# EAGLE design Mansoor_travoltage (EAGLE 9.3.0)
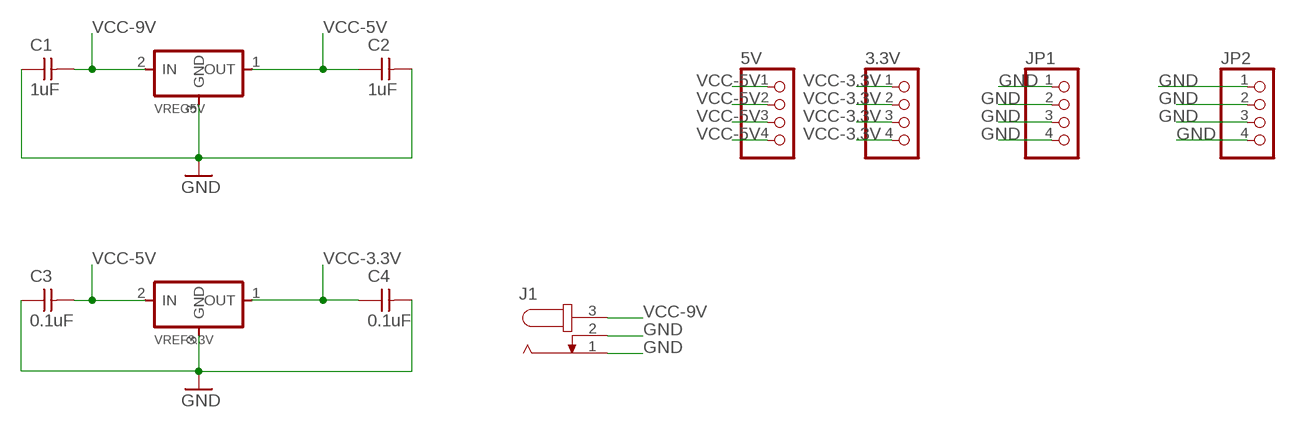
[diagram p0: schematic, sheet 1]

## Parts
3.3V  PINHD-1X4/LONG  [1X04]
5V  PINHD-1X4/LONG  [1X04]
C1  1uF  CAP-UNPOLARIZEDFAB  [C1206FAB]
C2  1uF  CAP-UNPOLARIZEDFAB  [C1206FAB]
C3  0.1uF  CAP-UNPOLARIZEDFAB  [C1206FAB]
C4  0.1uF  CAP-UNPOLARIZEDFAB  [C1206FAB]
J1  JACK-PLUG1  [SPC4078]
JP1  PINHD-1X4/LONG  [1X04]
JP2  PINHD-1X4/LONG  [1X04]
VREF3.3V  REGULATORSOT23  [SOT23]
VREG5V  REGULATORSOT23  [SOT23]

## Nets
GND: C1.1 C2.2 C3.1 C4.2 J1.1 J1.2 JP1.1 JP1.2 JP1.3 JP1.4 JP2.1 JP2.2 JP2.3 JP2.4 VREF3.3V.3(GND) VREG5V.3(GND)
VCC-3.3V: 3.3V.1 3.3V.2 3.3V.3 3.3V.4 C4.1 VREF3.3V.1(OUT)
VCC-5V: 5V.1 5V.2 5V.3 5V.4 C2.1 C3.2 VREF3.3V.2(IN) VREG5V.1(OUT)
VCC-9V: C1.2 J1.3 VREG5V.2(IN)

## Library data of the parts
3.3V 5V JP1 JP2 = pinhead_v2:PINHD-1X4: PIN HEADER
C1-C4 = fab:CAP-UNPOLARIZED
J1 = con-jack:JACK-PLUG: DC POWER JACK Power Jack, DC, Right Angle, Through Hole, Rated 5A at 16VDC, PC Terminals Distributor: Farnell (www.Farnell.de) Drawing: 84N1161.pdf / 84N1162.pdf Manufacturer: SPC Technology (www.spctechnology.com) Type: SPC4077 / SPC 4078; OC_FARNELL: unknown; OC_NEWARK: unknown
VREF3.3V VREG5V = fab:REGULATOR

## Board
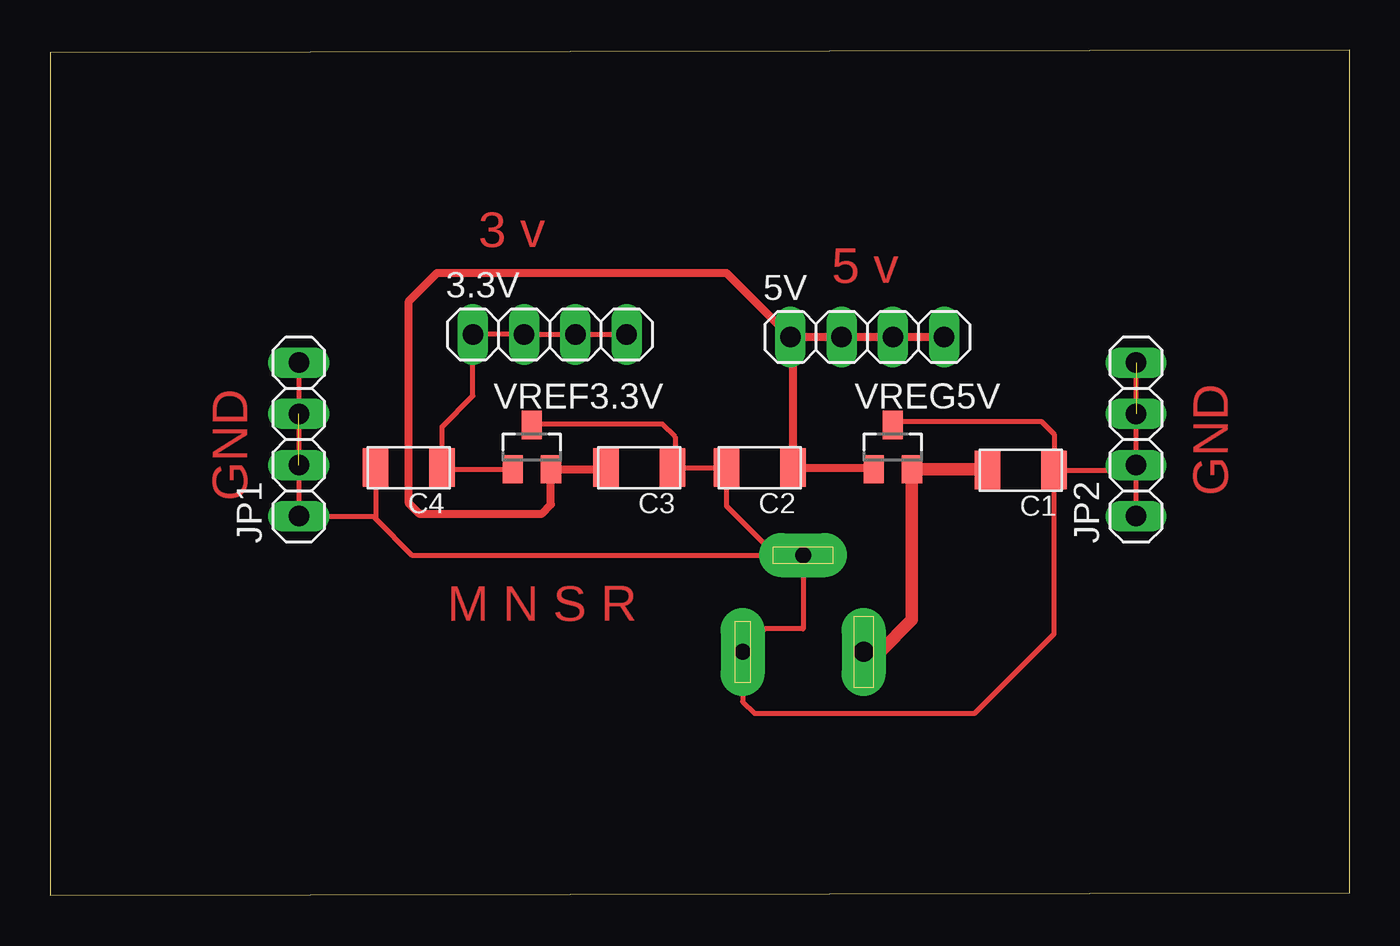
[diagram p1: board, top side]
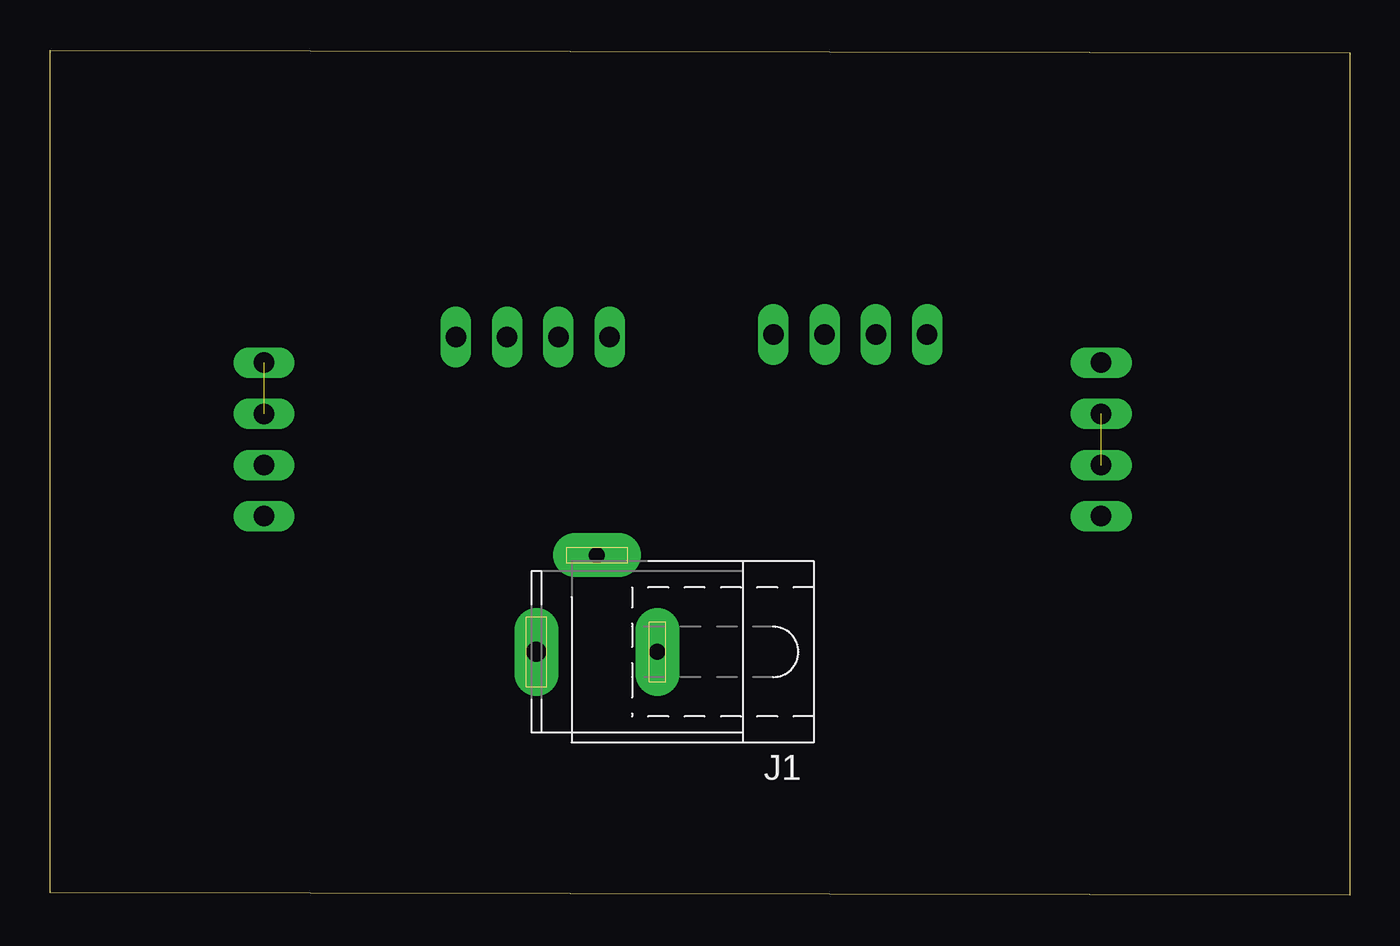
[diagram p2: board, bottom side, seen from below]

Size 64.44 x 41.9 mm. Coordinates in mm from the lower left corner, seen from the top.
Outline: 0,0 64.44,0.13 64.44,41.9 0,41.77 0,0
Copper layers (1*16): Top 0.035mm / dielectric 1.5mm / Bottom 0.035mm
Design rules "fabmodule": minimum track width 10mil, minimum drill 0.4mm, track to track 0.42mm, track to pad 0.42mm, pad to pad 0.42mm, via to via 0.42mm, smd to smd 0.42mm, copper to edge 40mil, drill to drill 0.8mm, minimum pad ring 10mil, minimum via ring 8mil, stop-mask expansion 4mil, vias tented up to drill 0mil, thermal gap 10mil

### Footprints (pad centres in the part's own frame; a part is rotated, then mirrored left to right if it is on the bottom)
1X04 = drill 1.016 long: 1 -3.81,0; 2 -1.27,0; 3 1.27,0; 4 3.81,0
C1206FAB = smd 1.27 x 1.905: 1 -1.651,0; 2 1.651,0
SPC4078 = drill 0.8 pad 2.184 long: 1 -3,0; 2 0,-4.8 | drill 1 pad 2.184 long: 3 3,0
SOT23 = smd 1 x 1.4: 1 -0.95,-1.1; 2 0.95,-1.1; 3 0,1.1

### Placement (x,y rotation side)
3.3V  24.77,27.81 0 top
5V  40.51,27.69 0 top
C1  48.13,21.08 180 top
C2  35.18,21.21 180 top
C3  29.21,21.21 180 top
C4  17.78,21.21 180 top
J1  37.34,12.06 180 bottom
JP1  12.32,22.61 90 top
JP2  53.85,22.61 90 top
VREF3.3V  23.88,22.23 0 top
VREG5V  41.78,22.23 0 top

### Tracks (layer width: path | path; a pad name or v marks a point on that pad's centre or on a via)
GND  (2 unrouted)
  Top 0.254: C4.2 16.13,18.8 | 16.13,18.8 16.13,18.67 17.93,16.87 J1.2 | J1.2 37.34,16.89 | VREG5V.3 41.95,23.49 49.15,23.49 49.78,22.86 C1.1 | VREF3.3V.3 23.92,23.37 30.35,23.37 30.99,22.73 30.99,21.34 C3.1 C2.2 33.53,19.3 35.97,16.87 J1.2 | J1.2 37.34,13.21 35.43,13.21 34.34,12.11 J1.1 34.34,9.6 34.93,9.02 45.85,9.02 49.78,12.95 C1.1 | 16.13,18.8 JP1.1 JP1.3 JP1.4 | C1.1 53.59,21.08 JP2.2 | JP2.1 JP2.2 | JP2.2 JP2.4
VCC-3.3V
  Top 0.254: VREF3.3V.1 19.52,21.12 C4.1 19.43,23.24 20.95,24.77 3.3V.1 3.3V.2 3.3V.3 3.3V.4
VCC-5V
  Top 0.254: 40.75,21.21 VREG5V.1 | 27.48,21.12 C3.2 | 36.83,27.69 5V.1 36.83,27.56
  Top 0.406: 40.75,21.21 C2.1 36.83,27.56 | 27.48,21.12 VREF3.3V.2 24.83,19.37 24.38,18.92 18.29,18.92 17.78,19.43 17.78,29.46 19.18,30.86 33.53,30.86 5V.1 | 36.83,27.69 5V.2 5V.3 5V.4
VCC-9V
  Top 0.254: 46.44,21.12 C1.2
  Top 0.61: J1.3 41.15,12.06 42.73,13.65 VREG5V.2 46.44,21.12

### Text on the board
Top: 3 v | 5 v | GND | GND | M N S R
